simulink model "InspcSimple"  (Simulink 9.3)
settings: Solver=FixedStepDiscrete  StartTime=0.0  StopTime=100000  FixedStep=Tstep  RelTol=1e-3  EnableMultiTasking=on
PreLoadFcn:
  | Test_LibVishia_Inspc.Test_LibVishia_Inspc_init();
InitFcn:
  | Test_LibVishia_Inspc.Test_LibVishia_Inspc_init();
libraries: libVishia_Inspc x3

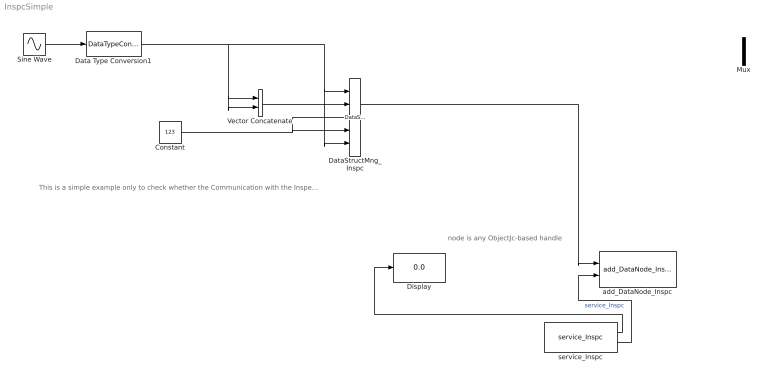
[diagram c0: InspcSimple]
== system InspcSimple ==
  note: This is a simple example only to check whether the Communication with the Inspector runs.
  note: node is any ObjectJc-based handle
  Constant : Constant  Value=123  OutDataTypeStr=int32
  Data Type Conversion1 : DataTypeConversion  OutDataTypeStr=single
  DataStructMng_Inspc : libVishia_Inspc/DataStructMng_Inspc  dirGenSource=''  typeData='TypeData'  inherit=off  chain=off  inputs=|
      | name;           //simple variable, type from connection 
      | name2: F*2;    //float[2] variable (single, type definded) 
      | =n3 :I, n4;     //2 int32 variables, only initialized 
      | -27 F5;           //Variable, type from connection, access rights set.
  Display : Display
  Mux : Mux  Inputs=2
  Sine Wave : Sin  SampleTime=0
  Vector Concatenate : Concatenate
  add_DataNode_Inspc : libVishia_Inspc/add_DataNode_Inspc  name1Refl='main'  name2Refl='_data'
  service_Inspc : libVishia_Inspc/service_Inspc  Tstep=Tstep  IpPort='UDP:0.0.0.0:60094'
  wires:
  service_Inspc/2 -> add_DataNode_Inspc/2  "service_Inspc"
  service_Inspc/1 -> Display/1
  DataStructMng_Inspc/1 -> add_DataNode_Inspc/1
  Vector Concatenate/1 -> DataStructMng_Inspc/2
  Sine Wave/1 -> Data Type Conversion1/1
  Data Type Conversion1/1 -> Vector Concatenate/2, Vector Concatenate/1, DataStructMng_Inspc/5, DataStructMng_Inspc/1
  Constant/1 -> DataStructMng_Inspc/3, DataStructMng_Inspc/4
